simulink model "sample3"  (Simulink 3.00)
settings: Solver=ode4  SolverMode=SingleTasking  StartTime=0.0  StopTime=60  FixedStep=0.2  MaxStep=0.04  RelTol=1e-3  AbsTol=1e-6

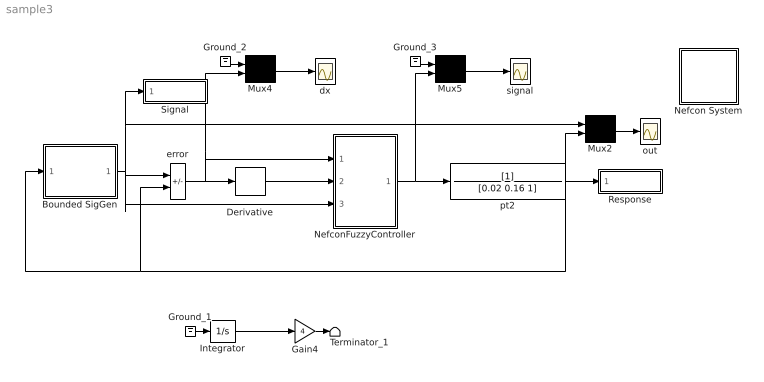
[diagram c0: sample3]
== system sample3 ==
  Bounded SigGen : Subsystem
  Derivative : Derivative
  Gain4 : Gain  Gain=4  SaturateOnIntegerOverflow=on
  Ground_1 : Ground
  Ground_2 : Ground
  Ground_3 : Ground
  Integrator : Integrator  ExternalReset=none  InitialConditionSource=internal  InitialCondition=0  LimitOutput=off  UpperSaturationLimit=inf  LowerSaturationLimit=-inf  ShowSaturationPort=off  ShowStatePort=off  AbsoluteTolerance=auto
  Mux2 : Mux  Inputs=2
  Mux4 : Mux  Inputs=2
  Mux5 : Mux  Inputs=2
  Nefcon System : Subsystem
  NefconFuzzyController : Subsystem
  Response : Subsystem
  Signal : Subsystem
  Terminator_1 : Terminator
  dx : Scope
  error : Sum  Inputs=+-  SaturateOnIntegerOverflow=on
  out : Scope
  pt2 : TransferFcn  Numerator=[1]  Denominator=[0.02 0.16 1]
  signal : Scope
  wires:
  Integrator/1 -> Gain4/1
  Bounded SigGen/1(out_1) -> Signal/1(In1), Mux2/1, NefconFuzzyController/3(in_3), error/1
  NefconFuzzyController/1(out_1) -> Mux5/2, pt2/1
  Mux5/1 -> signal/1
  Mux4/1 -> dx/1
  pt2/1 -> Bounded SigGen/1(in_1), error/2, Response/1(In1), Mux2/2
  error/1 -> NefconFuzzyController/1(in_1), Mux4/2, Derivative/1
  Derivative/1 -> NefconFuzzyController/2(in_2)
  Mux2/1 -> out/1
  Gain4/1 -> Terminator_1/1
  Ground_1/1 -> Integrator/1
  Ground_2/1 -> Mux4/1
  Ground_3/1 -> Mux5/1

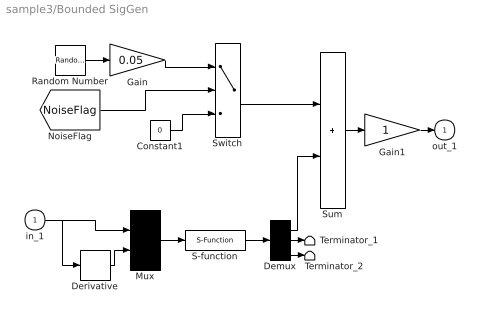
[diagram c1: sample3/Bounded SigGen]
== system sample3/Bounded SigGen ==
  in_1 : Inport  Port=1  PortWidth=-1  SampleTime=-1  DataType=auto
  Constant1 : Constant  Value=0
  Demux : Demux  Outputs=3
  Derivative : Derivative
  Gain : Gain  Gain=0.05  SaturateOnIntegerOverflow=on
  Gain1 : Gain  Gain=1  SaturateOnIntegerOverflow=on
  Mux : Mux  Inputs=2
  Random Number : RandomNumber  Mean=0  Variance=1  Seed=0  SampleTime=0
  S-function : S-Function  FunctionName=snefsign  PortCounts=[]  SFunctionModules=''
  Sum : Sum  Inputs=++  SaturateOnIntegerOverflow=on
  Switch : Switch  Threshold=0.5
  Terminator_1 : Terminator
  Terminator_2 : Terminator
  out_1 : Outport  Port=1
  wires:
  [NoiseFlag] -> Switch/2
  Gain1/1 -> out_1/1
  Sum/1 -> Gain1/1
  Switch/1 -> Sum/1
  Constant1/1 -> Switch/3
  Gain/1 -> Switch/1
  Random Number/1 -> Gain/1
  Demux/1 -> Sum/2
  S-function/1 -> Demux/1
  Mux/1 -> S-function/1
  Derivative/1 -> Mux/2
  in_1/1 -> Mux/1, Derivative/1
  Demux/2 -> Terminator_1/1
  Demux/3 -> Terminator_2/1

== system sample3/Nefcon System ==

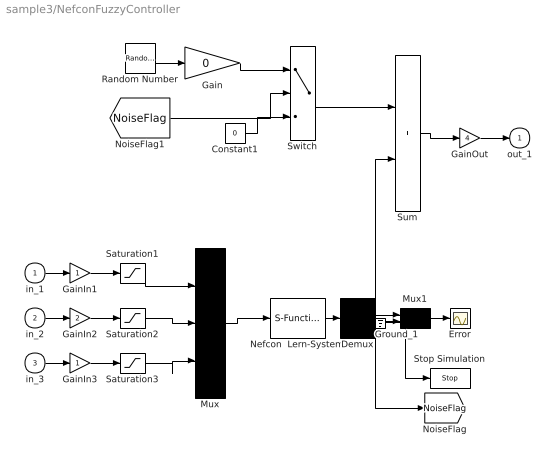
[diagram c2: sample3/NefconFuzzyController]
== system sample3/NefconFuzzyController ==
  in_1 : Inport  Port=1  PortWidth=-1  SampleTime=-1  DataType=auto
  in_2 : Inport  Port=2  PortWidth=-1  SampleTime=-1  DataType=auto
  in_3 : Inport  Port=3  PortWidth=-1  SampleTime=-1  DataType=auto
  Constant1 : Constant  Value=0
  Demux : Demux  Outputs=4
  Error : Scope
  Gain : Gain  Gain=0  SaturateOnIntegerOverflow=on
  GainIn1 : Gain  Gain=1  SaturateOnIntegerOverflow=on
  GainIn2 : Gain  Gain=2  SaturateOnIntegerOverflow=on
  GainIn3 : Gain  Gain=1  SaturateOnIntegerOverflow=on
  GainOut : Gain  Gain=4  SaturateOnIntegerOverflow=on
  Ground_1 : Ground
  Mux : Mux  Inputs=3
  Mux1 : Mux  Inputs=2
  Nefcon  Lern-System : S-Function  FunctionName=snefcon  PortCounts=[]  SFunctionModules=''
  Random Number : RandomNumber  Mean=0  Variance=1  Seed=0  SampleTime=0
  Saturation1 : Saturate  UpperLimit=1  LowerLimit=-1
  Saturation2 : Saturate  UpperLimit=1  LowerLimit=-1
  Saturation3 : Saturate  UpperLimit=1  LowerLimit=-1
  Stop Simulation : Stop
  Sum : Sum  Inputs=++  SaturateOnIntegerOverflow=on
  Switch : Switch  Threshold=0.5
  out_1 : Outport  Port=1
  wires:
  Demux/4 -> [NoiseFlag]
  Demux/1 -> Sum/2
  Sum/1 -> GainOut/1
  Random Number/1 -> Gain/1
  Gain/1 -> Switch/1
  Constant1/1 -> Switch/3
  Switch/1 -> Sum/1
  Demux/3 -> Stop Simulation/1
  Mux1/1 -> Error/1
  Demux/2 -> Mux1/1
  GainOut/1 -> out_1/1
  Nefcon  Lern-System/1 -> Demux/1
  Mux/1 -> Nefcon  Lern-System/1
  Saturation3/1 -> Mux/3
  GainIn3/1 -> Saturation3/1
  in_3/1 -> GainIn3/1
  Saturation2/1 -> Mux/2
  GainIn2/1 -> Saturation2/1
  in_2/1 -> GainIn2/1
  Saturation1/1 -> Mux/1
  GainIn1/1 -> Saturation1/1
  in_1/1 -> GainIn1/1
  [NoiseFlag] -> Switch/2
  Ground_1/1 -> Mux1/2

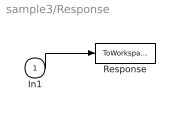
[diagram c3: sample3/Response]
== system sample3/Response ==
  In1 : Inport  Port=1  PortWidth=-1  SampleTime=-1  DataType=auto
  Response : ToWorkspace  VariableName=nef_y  SampleTime=0  SaveFormat=Matrix
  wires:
  In1/1 -> Response/1

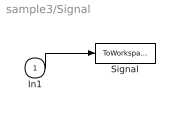
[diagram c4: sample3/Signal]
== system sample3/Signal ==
  In1 : Inport  Port=1  PortWidth=-1  SampleTime=-1  DataType=auto
  Signal : ToWorkspace  VariableName=nef_u  SampleTime=0  SaveFormat=Matrix
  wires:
  In1/1 -> Signal/1
